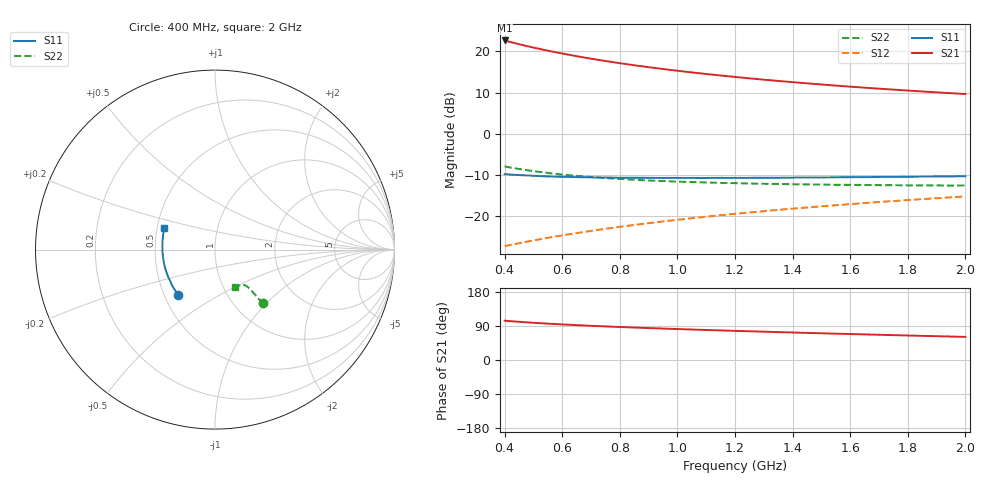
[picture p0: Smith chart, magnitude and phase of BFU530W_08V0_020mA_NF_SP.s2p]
! Filename:  P:\Prog\Test\Noise\ATS_data\Testdata_Net\06 Compressed Noise after Statistics\BFU530W_APM2013_09_A05_08p0V_020mA_NF_CM01_D.sf
! Date/Time: Tue 26/Mar/2013 18:06:03
! BFU530W_APM2013_09_A05_08p0V_1to25mA_NF_CM01_Bias8_R.sf
! Noise Parameter Data File
! BFU530W_APM2013_09_A05_08p0V_1to25mA_NF_CM01
! Date/time: Thu Mar 21 21:44:48 2013
! VAR V_out= 8.001000
! VAR I_out= 20.000000
! VAR V_in= 0.807700
! VAR I_in= 0.202100
! Device data file deembeded for feedlines and parallel
! Original file: \06 Compressed Noise after Statistics\BFU530W_APM2013_09_A05_08p0V_020mA_NF_CM01_R.sf
! Feed-files: PR019V01_070313_Feed1.s2p, PR019V01_070313_Feed2.s2p
! Parallel-file: PR019V01_070313_Par.s2p
# MHz S MA R 50
!  Freq-MHz  S11-mag  S11-arg  S21-mag  S21-arg  S12-mag  S12-arg  S22-mag  S22-arg
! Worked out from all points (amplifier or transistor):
!   37 points, 400 MHz to 2 GHz, reference 50 ohm
!   highest |S21| = 22.6 dB at 400 MHz (marker M1)
!   |S21| within 3 dB of that: start of sweep to 588.2 MHz
!   unconditionally stable (mu >= 1): 1.094 GHz to end of sweep
!   at 500 MHz: K = 0.87, MSG = 23.4 dB, |S12| = -25.8 dB
!   at 1.1 GHz: K = 1.00, MAG = 17.1 dB, |S12| = -20.1 dB
!   at 2 GHz: K = 1.01, MAG = 11.8 dB, |S12| = -15.2 dB
!   lowest NFmin = 0.99 dB at 433 MHz
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400  0.3254 -128.8  13.54 103.7  0.04362 65.5  0.4029 -48.0
420  0.3219 -131.5  12.98 102.5  0.04512 65.8  0.3912 -48.2
433  0.319 -133.2  12.63 101.8  0.04609 66.0  0.384 -48.3
460  0.3159 -136.2  11.97 100.3  0.04814 66.4  0.3713 -48.4
500  0.3109 -140.6  11.1 98.2  0.05112 66.9  0.3535 -48.4
550  0.3045 -145.1  10.19 95.9  0.05506 67.5  0.3363 -48.4
600  0.3024 -149.4  9.41 93.9  0.05895 68.0  0.3213 -48.4
650  0.2993 -153.2  8.734 92.0  0.06283 68.4  0.31 -48.4
700  0.2972 -156.8  8.147 90.2  0.0668 68.8  0.3 -48.5
750  0.296 -159.8  7.635 88.7  0.07078 69.2  0.2912 -48.4
800  0.2943 -162.8  7.184 87.1  0.0748 69.4  0.2849 -48.7
850  0.294 -165.6  6.785 85.7  0.0788 69.6  0.2779 -48.8
950  0.2924 -170.3  6.107 83.0  0.08698 69.9  0.2685 -49.2
1050  0.2926 -174.7  5.554 80.4  0.09513 70.0  0.2611 -49.8
1150  0.2935 -178.8  5.093 78.0  0.1033 70.0  0.2547 -50.6
1200  0.2929 179.5  4.895 76.9  0.1076 69.9  0.2531 -51.2
1250  0.2935 177.7  4.706 75.8  0.1116 69.8  0.2503 -51.6
1350  0.2944 174.5  4.38 73.6  0.1201 69.6  0.2474 -52.7
1500  0.2967 169.8  3.966 70.5  0.1325 69.0  0.2433 -54.8
1650  0.2991 165.5  3.627 67.6  0.1451 68.5  0.2401 -56.8
1750  0.3013 163.0  3.439 65.6  0.1536 68.0  0.2392 -58.3
2000  0.307 156.8  3.04 61.0  0.1746 66.6  0.237 -62.7
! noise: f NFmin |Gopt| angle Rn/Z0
400  1.026  0.232  -175.5  0.0807
460  1.046  0.2348  -174.4  0.0793
600  1.06  0.2221  -171.3  0.085
800  1.087  0.2525  -167.6  0.0794
1000  1.104  0.2635  -164.5  0.079
1200  1.119  0.276  -160.4  0.0827
1400  1.175  0.2894  -156.7  0.0812
1600  1.192  0.2971  -155.8  0.082
1800  1.195  0.3241  -149.7  0.0842
2000  1.217  0.3448  -147.1  0.087
